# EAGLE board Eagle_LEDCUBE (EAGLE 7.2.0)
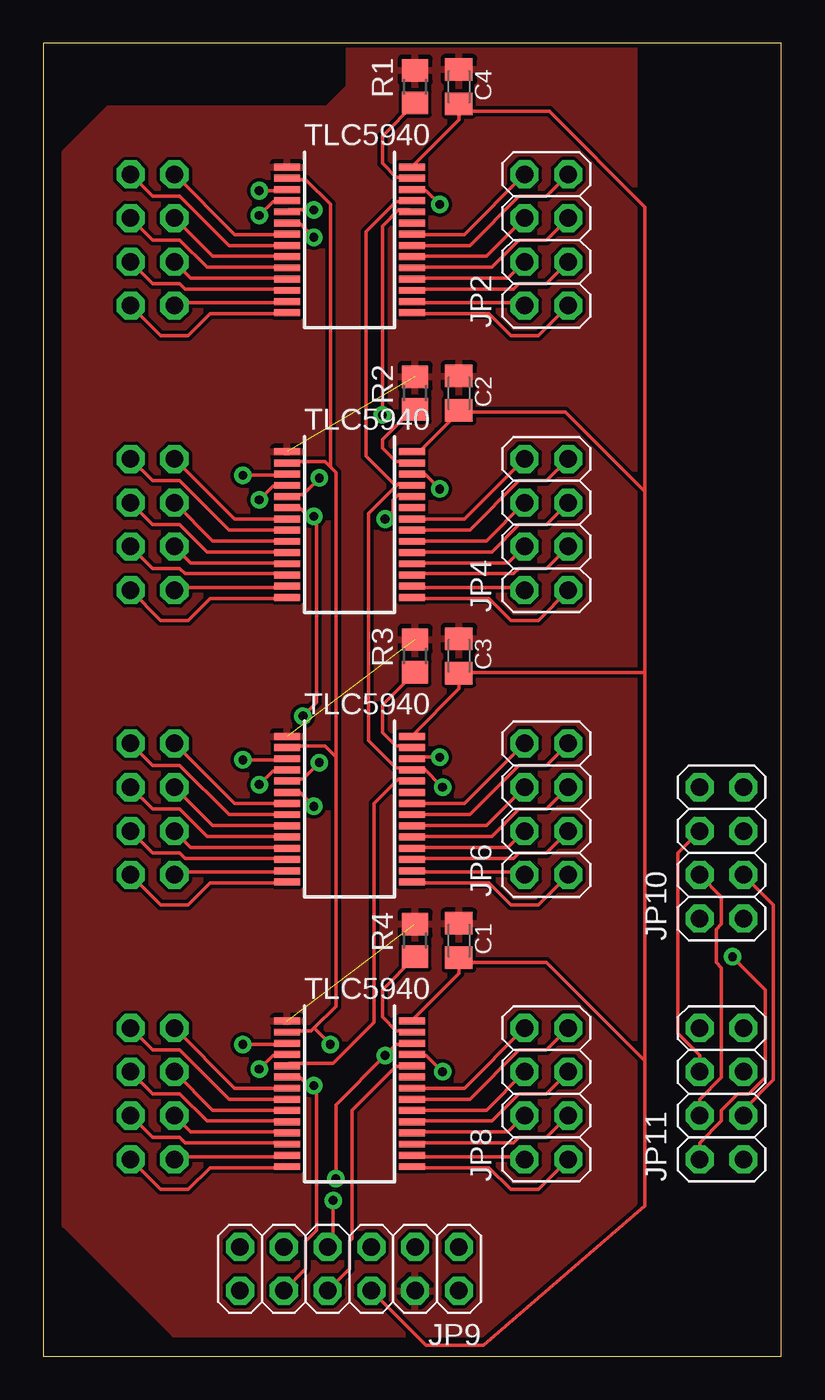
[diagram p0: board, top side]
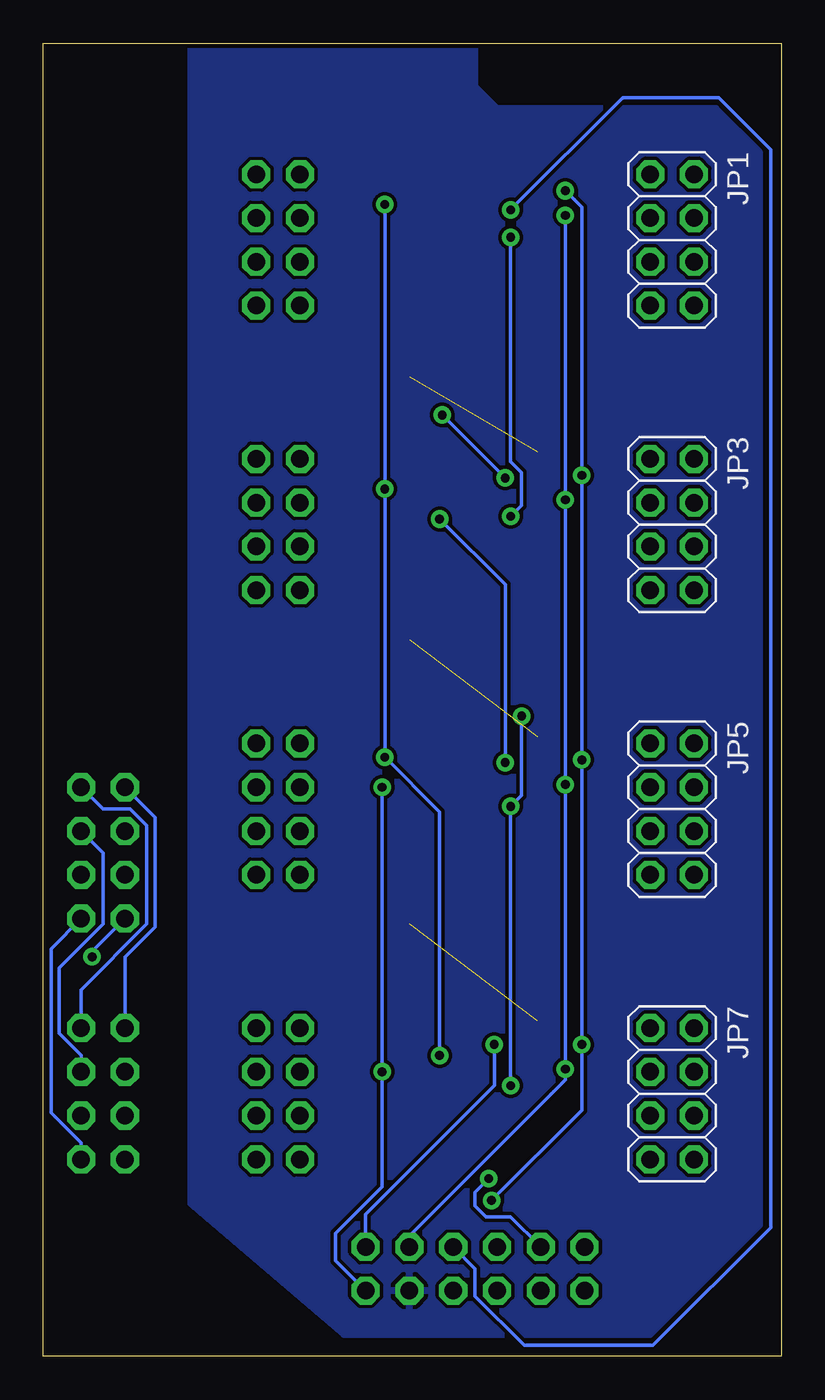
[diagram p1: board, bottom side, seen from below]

Size 42.85 x 76.19 mm. Coordinates in mm from the lower left corner, seen from the top.
Outline: 0,0 42.85,0 42.85,76.19 0,76.19 0,0
Copper layers (1*16): Top 0.035mm / dielectric 1.5mm / Bottom 0.035mm
Design rules "8mils": minimum track width 8mil, minimum drill 20mil, track to track 8mil, track to pad 8mil, pad to pad 8mil, via to via 8mil, smd to smd 8mil, copper to edge 10mil, drill to drill 8mil, minimum pad ring 12mil, minimum via ring 10mil, stop-mask expansion 4mil, vias tented up to drill 25mil, thermal gap 10mil

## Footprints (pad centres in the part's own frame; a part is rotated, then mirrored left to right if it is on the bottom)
C0805K = smd 1.3 x 1.6: 1 -1,0; 2 1,0
IC-SSOP28 = smd 0.4 x 1.5: 1 -4.225,-3.625; 2 -3.575,-3.625; 3 -2.925,-3.625; 4 -2.275,-3.625; 5 -1.625,-3.625; 6 -0.975,-3.625; 7 -0.325,-3.625; 8 0.325,-3.625; 9 0.975,-3.625; 10 1.625,-3.625; 11 2.275,-3.625; 12 2.925,-3.625; 13 3.575,-3.625; 14 4.225,-3.625; 15 4.225,3.625; 16 3.575,3.625; 17 2.925,3.625; 18 2.275,3.625; 19 1.625,3.625; 20 0.975,3.625; 21 0.325,3.625; 22 -0.325,3.625; 23 -0.975,3.625; 24 -1.625,3.625; 25 -2.275,3.625; 26 -2.925,3.625; 27 -3.575,3.625; 28 -4.225,3.625
2X04 = drill 1.016 octagon: 1 -3.81,-1.27; 2 -3.81,1.27; 3 -1.27,-1.27; 4 -1.27,1.27; 5 1.27,-1.27; 6 1.27,1.27; 7 3.81,-1.27; 8 3.81,1.27
2X06 = drill 1.016 octagon: 1 -6.35,-1.27; 2 -6.35,1.27; 3 -3.81,-1.27; 4 -3.81,1.27; 5 -1.27,-1.27; 6 -1.27,1.27; 7 1.27,-1.27; 8 1.27,1.27; 9 3.81,-1.27; 10 3.81,1.27; 11 6.35,-1.27; 12 6.35,1.27
R0805 = smd 1.3 x 1.5: 1 -0.95,0; 2 0.95,0

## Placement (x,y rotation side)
C1  [C0805K]  24.13,24.13 270 top
C2  [C0805K]  24.13,55.88 270 top
C3  [C0805K]  24.13,40.64 270 top
C4  [C0805K]  24.13,73.66 270 top
IC1  [IC-SSOP28]  17.78,64.77 270 top
IC2  [IC-SSOP28]  17.78,48.26 270 top
IC3  [IC-SSOP28]  17.78,31.75 270 top
IC4  [IC-SSOP28]  17.78,15.24 270 top
JP1  [2X04]  6.35,64.77 270 bottom
JP2  [2X04]  29.21,64.77 90 top
JP3  [2X04]  6.35,48.26 270 bottom
JP4  [2X04]  29.21,48.26 90 top
JP5  [2X04]  6.35,31.75 270 bottom
JP6  [2X04]  29.21,31.75 90 top
JP7  [2X04]  6.35,15.24 270 bottom
JP8  [2X04]  29.21,15.24 90 top
JP9  [2X06]  17.78,5.08 180 top
JP10  [2X04]  39.37,29.21 90 top
JP11  [2X04]  39.37,15.24 90 top
R1  2.2k  [R0805]  21.59,73.66 90 top
R2  2.2k  [R0805]  21.59,55.88 90 top
R3  2.2k  [R0805]  21.59,40.64 90 top
R4  2.2k  [R0805]  21.59,24.13 90 top

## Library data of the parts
C1-C4 R1-R4 = resistor
IC1-IC4 = TLC5940
JP1-JP11 = pinhead

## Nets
A1: IC1.7 JP1.1
A2: IC1.8 JP1.2
A3: IC1.9 JP1.3
A4: IC1.10 JP1.4
A5: IC1.11 JP1.5
A6: IC1.12 JP1.6
A7: IC1.13 JP1.7
A8: IC1.14 JP1.8
A9: IC1.15 JP2.1
A10: IC1.16 JP2.2
A11: IC1.17 JP2.3
A12: IC1.18 JP2.4
A13: IC1.19 JP2.5
A14: IC1.20 JP2.6
A15: IC1.21 JP2.7
A16: IC1.22 JP2.8
B1: IC2.7 JP3.1
B2: IC2.8 JP3.2
B3: IC2.9 JP3.3
B4: IC2.10 JP3.4
B5: IC2.11 JP3.5
B6: IC2.12 JP3.6
B7: IC2.13 JP3.7
B8: IC2.14 JP3.8
B9: IC2.15 JP4.1
B10: IC2.16 JP4.2
B11: IC2.17 JP4.3
B12: IC2.18 JP4.4
B13: IC2.19 JP4.5
B14: IC2.20 JP4.6
B15: IC2.21 JP4.7
B16: IC2.22 JP4.8
BLANK: IC1.2 IC2.2 IC3.2 IC4.2 JP9.1
C1: IC3.7 JP5.1
C2: IC3.8 JP5.2
C3: IC3.9 JP5.3
C4: IC3.10 JP5.4
C5: IC3.11 JP5.5
C6: IC3.12 JP5.6
C7: IC3.13 JP5.7
C8: IC3.14 JP5.8
C9: IC3.15 JP6.1
C10: IC3.16 JP6.2
C11: IC3.17 JP6.3
C12: IC3.18 JP6.4
C13: IC3.19 JP6.5
C14: IC3.20 JP6.6
C15: IC3.21 JP6.7
C16: IC3.22 JP6.8
D1: IC4.7 JP7.1
D2: IC4.8 JP7.2
D3: IC4.9 JP7.3
D4: IC4.10 JP7.4
D5: IC4.11 JP7.5
D6: IC4.12 JP7.6
D7: IC4.13 JP7.7
D8: IC4.14 JP7.8
D9: IC4.15 JP8.1
D10: IC4.16 JP8.2
D11: IC4.17 JP8.3
D12: IC4.18 JP8.4
D13: IC4.19 JP8.5
D14: IC4.20 JP8.6
D15: IC4.21 JP8.7
D16: IC4.22 JP8.8
DCPRG: IC1.26 IC2.26 IC3.26 IC4.26 JP9.9
GND: C1.1 C2.1 C3.1 C4.1 IC1.1 IC2.1 IC3.1 IC4.1 JP9.4 R1.2 R2.2 R3.2 R4.2
GSCLK: IC1.25 IC2.25 IC3.25 IC4.25 JP9.2
L1: JP10.1 JP11.1
L2: JP10.2 JP11.2
L3: JP10.3 JP11.3
L4: JP10.4 JP11.4
L5: JP10.5 JP11.5
L6: JP10.6 JP11.6
L7: JP10.7 JP11.7
L8: JP10.8 JP11.8
N$5: IC1.27 R1.1
N$16: IC2.27 R2.1
N$26: IC3.27 R3.1
N$35: IC4.27 R4.1
SCLK: IC1.4 IC2.4 IC3.4 IC4.4 JP9.3
SIN: IC1.5 JP9.5
SIN_B: IC1.24 IC2.5
SIN_C: IC2.24 IC3.5
SIN_D: IC3.24 IC4.5
SIN_E: IC4.24 JP9.8
VCC: C1.2 C2.2 C3.2 C4.2 IC1.28 IC2.28 IC3.28 IC4.28 JP9.6
VPRG: IC1.6 IC2.6 IC3.6 IC4.6 JP9.10
XLAT: IC1.3 IC2.3 IC3.3 IC4.3 JP9.7

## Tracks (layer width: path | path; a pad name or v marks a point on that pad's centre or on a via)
A1
  Top 0.203: JP1.1 11.11,65.09 14.13,65.09 IC1.7
A2
  Top 0.203: JP1.2 6.35,67.31 7.94,67.31 10.79,64.45 14.13,64.45 IC1.8
A3
  Top 0.203: JP1.3 9.84,63.82 14.13,63.82 IC1.9
A4
  Top 0.203: JP1.4 6.35,64.77 7.94,64.77 9.52,63.18 14.13,63.18 IC1.10
A5
  Top 0.203: JP1.5 8.57,62.55 14.13,62.55 IC1.11
A6
  Top 0.203: JP1.6 6.35,62.23 7.94,62.23 8.25,61.91 14.13,61.91 IC1.12
A7
  Top 0.203: JP1.7 7.78,61.12 14.13,61.12 IC1.13
A8
  Top 0.203: JP1.8 6.83,59.21 8.41,59.21 9.68,60.48 14.13,60.48 IC1.14
A9
  Top 0.203: JP2.1 28.73,59.21 27.15,59.21 25.88,60.48 21.43,60.48 IC1.15
A10
  Top 0.203: JP2.2 27.78,61.12 21.43,61.12 IC1.16
A11
  Top 0.203: JP2.3 29.21,62.23 27.62,62.23 27.31,61.91 21.43,61.91 IC1.17
A12
  Top 0.203: JP2.4 26.99,62.55 21.43,62.55 IC1.18
A13
  Top 0.203: JP2.5 29.21,64.77 27.62,64.77 26.04,63.18 21.43,63.18 IC1.19
A14
  Top 0.203: JP2.6 25.72,63.82 21.43,63.82 IC1.20
A15
  Top 0.203: JP2.7 29.21,67.31 27.62,67.31 24.76,64.45 21.43,64.45 IC1.21
A16
  Top 0.203: JP2.8 24.45,65.09 21.43,65.09 IC1.22
B1
  Top 0.203: JP3.1 11.11,48.58 14.13,48.58 IC2.7
B2
  Top 0.203: JP3.2 6.35,50.8 7.94,50.8 10.79,47.94 14.13,47.94 IC2.8
B3
  Top 0.203: JP3.3 9.84,47.31 14.13,47.31 IC2.9
B4
  Top 0.203: JP3.4 6.35,48.26 7.94,48.26 9.52,46.67 14.13,46.67 IC2.10
B5
  Top 0.203: JP3.5 8.57,46.04 14.13,46.04 IC2.11
B6
  Top 0.203: JP3.6 6.35,45.72 7.94,45.72 8.25,45.4 14.13,45.4 IC2.12
B7
  Top 0.203: JP3.7 7.78,44.61 14.13,44.61 IC2.13
B8
  Top 0.203: JP3.8 6.83,42.7 8.41,42.7 9.68,43.97 14.13,43.97 IC2.14
B9
  Top 0.203: JP4.1 28.73,42.7 27.15,42.7 25.88,43.97 21.43,43.97 IC2.15
B10
  Top 0.203: JP4.2 27.78,44.61 21.43,44.61 IC2.16
B11
  Top 0.203: JP4.3 29.21,45.72 27.62,45.72 27.31,45.4 21.43,45.4 IC2.17
B12
  Top 0.203: JP4.4 26.99,46.04 21.43,46.04 IC2.18
B13
  Top 0.203: JP4.5 29.21,48.26 27.62,48.26 26.04,46.67 21.43,46.67 IC2.19
B14
  Top 0.203: JP4.6 25.72,47.31 21.43,47.31 IC2.20
B15
  Top 0.203: JP4.7 29.21,50.8 27.62,50.8 24.76,47.94 21.43,47.94 IC2.21
B16
  Top 0.203: JP4.8 24.45,48.58 21.43,48.58 IC2.22
BLANK  (via drill 0.51)
  Top 0.203: 15.72,19.05 16.99,20.32 16.99,34.77 | 15.72,19.05 15.56,18.89 14.29,18.89 IC4.2 | 16.99,34.77 16.35,35.4 14.29,35.4 IC3.2 | 16.67,51.59 16.99,51.28 16.99,34.77 | 16.67,51.59 16.35,51.91 14.29,51.91 IC2.2 | 16.67,51.59 16.67,66.83 15.24,68.26 14.29,68.26 IC1.2 | 15.72,19.05 v16.67,18.1
  Bottom 0.203: JP9.1 24.13,8.26 16.67,15.72 v16.67,18.1
C1
  Top 0.203: JP5.1 11.11,32.07 14.13,32.07 IC3.7
C2
  Top 0.203: JP5.2 6.35,34.29 7.94,34.29 10.79,31.43 14.13,31.43 IC3.8
C3
  Top 0.203: JP5.3 9.84,30.8 14.13,30.8 IC3.9
C4
  Top 0.203: JP5.4 6.35,31.75 7.94,31.75 9.52,30.16 14.13,30.16 IC3.10
C5
  Top 0.203: JP5.5 8.57,29.53 14.13,29.53 IC3.11
C6
  Top 0.203: JP5.6 6.35,29.21 7.94,29.21 8.25,28.89 14.13,28.89 IC3.12
C7
  Top 0.203: JP5.7 7.78,28.1 14.13,28.1 IC3.13
C8
  Top 0.203: JP5.8 6.83,26.19 8.41,26.19 9.68,27.46 14.13,27.46 IC3.14
C9
  Top 0.203: JP6.1 28.73,26.19 27.15,26.19 25.88,27.46 21.43,27.46 IC3.15
C10
  Top 0.203: JP6.2 27.78,28.1 21.43,28.1 IC3.16
C11
  Top 0.203: JP6.3 29.21,29.21 27.62,29.21 27.31,28.89 21.43,28.89 IC3.17
C12
  Top 0.203: JP6.4 26.99,29.53 21.43,29.53 IC3.18
C13
  Top 0.203: JP6.5 29.21,31.75 27.62,31.75 26.04,30.16 21.43,30.16 IC3.19
C14
  Top 0.203: JP6.6 25.72,30.8 21.43,30.8 IC3.20
C15
  Top 0.203: JP6.7 29.21,34.29 27.62,34.29 24.76,31.43 21.43,31.43 IC3.21
C16
  Top 0.203: JP6.8 24.45,32.07 21.43,32.07 IC3.22
D1
  Top 0.203: JP7.1 11.11,15.56 14.13,15.56 IC4.7
D2
  Top 0.203: JP7.2 6.35,17.78 7.94,17.78 10.79,14.92 14.13,14.92 IC4.8
D3
  Top 0.203: JP7.3 9.84,14.29 14.13,14.29 IC4.9
D4
  Top 0.203: JP7.4 6.35,15.24 7.94,15.24 9.52,13.65 14.13,13.65 IC4.10
D5
  Top 0.203: JP7.5 8.57,13.02 14.13,13.02 IC4.11
D6
  Top 0.203: JP7.6 6.35,12.7 7.94,12.7 8.25,12.38 14.13,12.38 IC4.12
D7
  Top 0.203: JP7.7 7.78,11.59 14.13,11.59 IC4.13
D8
  Top 0.203: JP7.8 6.83,9.68 8.41,9.68 9.68,10.95 14.13,10.95 IC4.14
D9
  Top 0.203: JP8.1 28.73,9.68 27.15,9.68 25.88,10.95 21.43,10.95 IC4.15
D10
  Top 0.203: JP8.2 27.78,11.59 21.43,11.59 IC4.16
D11
  Top 0.203: JP8.3 29.21,12.7 27.62,12.7 27.31,12.38 21.43,12.38 IC4.17
D12
  Top 0.203: JP8.4 26.99,13.02 21.43,13.02 IC4.18
D13
  Top 0.203: JP8.5 29.21,15.24 27.62,15.24 26.04,13.65 21.43,13.65 IC4.19
D14
  Top 0.203: JP8.6 25.72,14.29 21.43,14.29 IC4.20
D15
  Top 0.203: JP8.7 29.21,17.78 27.62,17.78 24.76,14.92 21.43,14.92 IC4.21
D16
  Top 0.203: JP8.8 24.45,15.56 21.43,15.56 IC4.22
DCPRG  (via drill 0.51)
  Top 0.203: v16.99,10.32 16.99,14.61 v19.84,17.46 20.48,18.1 21.27,18.1 IC4.26 | v23.02,34.77 21.43,34.77 IC3.26 | v23.02,50.32 22.07,51.28 21.43,51.28 IC2.26 | v23.02,66.83 22.22,67.63 21.43,67.63 IC1.26
  Bottom 0.203: v16.99,10.32 17.78,9.53 17.78,8.73 17.14,8.1 15.72,8.1 JP9.9 | v23.02,66.83 v23.02,50.32 v23.02,34.77 19.84,31.59 v19.84,17.46
GND  (3 unrouted)
  pour Bottom: 1.27,7.62 1.27,69.85 3.81,72.39 16.51,72.39 17.78,73.66 17.78,76.2 34.29,76.2 34.29,8.89 25.4,1.27 7.62,1.27
  pour Top: 1.27,7.62 1.27,69.85 3.81,72.39 16.51,72.39 17.78,73.66 17.78,76.2 34.29,76.2 34.29,8.89 25.4,1.27 7.62,1.27
GSCLK  (via drill 0.51)
  Top 0.203: v23.18,16.51 22.22,17.46 21.43,17.46 IC4.25 | 20.48,50.48 20.64,50.64 21.27,50.64 IC2.25 | 20.48,50.48 18.89,48.9 18.89,35.72 20.48,34.13 21.27,34.13 IC3.25 21.43,34.13 22.07,34.13 v23.18,33.02 | 20.48,50.48 18.73,52.23 18.73,65.25 20.48,66.99 21.27,66.99 IC1.25
  Bottom 0.203: JP9.2 25.88,5.56 25.88,7.14 23.18,9.84 v23.18,16.51 v23.18,33.02
L1
  Bottom 0.203: JP11.1 40.64,12.38 42.39,14.13 42.39,23.65 JP10.1
L2  (via drill 0.51)
  Top 0.203: JP11.2 38.1,12.38 39.37,13.65 39.37,14.29 40.32,15.24 40.96,15.24 41.91,16.19 41.91,21.27 v40,23.18
  Bottom 0.203: v40,23.18 40,23.5 JP10.2
L3
  Top 0.203: JP11.3 40.64,14.29 42.39,16.03 42.39,26.19 JP10.3
L4
  Top 0.203: JP11.4 38.1,14.92 39.37,16.19 39.37,22.54 39.05,22.86 39.05,24.77 39.37,25.08 39.37,26.67 JP10.4
L5
  Bottom 0.203: JP11.5 40.64,17.46 41.91,18.73 41.91,22.54 39.37,25.08 39.37,29.21 JP10.5
L6
  Top 0.203: JP11.6 38.1,17.46 36.83,18.73 36.83,29.21 JP10.6
L7
  Bottom 0.203: JP11.7 40.64,21.27 36.83,25.08 36.83,30.8 37.78,31.75 39.37,31.75 JP10.7
L8
  Bottom 0.203: JP11.8 38.1,23.18 36.35,24.92 36.35,31.27 JP10.8
N$5
  Top 0.203: IC1.27 21.27,68.42 20.48,68.42 19.68,69.22 19.68,70.8 R1.1
N$16
  Top 0.203: IC2.27 21.27,51.91 20.48,51.91 19.68,52.7 19.68,53.18 21.59,55.09 R2.1
N$26
  Top 0.203: IC3.27 21.27,35.4 20.48,35.4 19.68,36.2 19.68,37.78 R3.1
N$35
  Top 0.203: IC4.27 21.27,18.89 20.48,18.89 19.68,19.68 19.68,21.27 R4.1
SCLK  (via drill 0.51)
  Top 0.203: v12.54,16.67 13.34,17.46 14.13,17.46 IC4.4 | v12.54,33.18 13.34,33.97 14.13,33.97 IC3.4 | v12.54,49.69 13.34,50.48 14.13,50.48 IC2.4 | v12.54,66.2 13.34,66.99 14.13,66.99 IC1.4
  Bottom 0.203: JP9.3 21.59,6.99 12.54,16.03 v12.54,16.67 v12.54,33.18 v12.54,49.69 v12.54,66.2
SIN  (via drill 0.51)
  Top 0.203: v15.72,66.52 14.29,66.52 IC1.5
  Bottom 0.203: v15.72,66.52 9.21,73.03 3.65,73.03 0.63,70.01 0.63,7.46 7.46,0.64 14.92,0.64 17.78,3.49 17.78,5.08 JP9.5
SIN_B  (via drill 0.51)
  Top 0.203: v16.03,50.96 15.08,50.01 14.29,50.01 IC2.5 | v19.68,54.61 19.68,65.56 20.64,66.52 21.27,66.52 IC1.24
  Bottom 0.203: v19.68,54.61 v16.03,50.96
SIN_C  (via drill 0.51)
  Top 0.203: v16.03,34.45 15.08,33.5 14.29,33.5 IC3.5 | v19.84,48.58 20.32,49.05 20.32,49.69 20.64,50.01 21.27,50.01 IC2.24
  Bottom 0.203: v16.03,34.45 16.03,44.77 v19.84,48.58
SIN_D
  Top 0.203: IC4.5 14.29,16.99 16.83,16.99 19.21,19.37 19.21,32.07 20.64,33.5 21.27,33.5 IC3.24
SIN_E
  Top 0.203: JP9.8 17.78,5.08 17.78,6.67 17.94,6.83 17.94,14.29 20.48,16.83 21.27,16.83 IC4.24
VCC
  Top 0.203: 24.13,72.23 C4.2 24.13,72.55 | 24.13,72.23 24.13,71.75 21.43,69.06 IC1.28 | IC3.28 21.43,36.04 24.13,38.73 C3.2 24.13,39.69 34.92,39.69 | 24.13,54.77 21.91,52.55 21.43,52.55 IC2.28 | 24.13,22.86 C1.2 24.13,23.02 | 24.13,22.86 24.13,22.23 21.43,19.53 IC4.28 | JP9.6 22.22,0.64 25.56,0.64 34.92,8.73 34.92,17.14 | 34.92,17.14 29.21,22.86 24.13,22.86 | 24.13,54.77 30.32,54.77 34.92,50.16 | 34.92,17.14 34.92,39.69 | 34.92,39.69 34.92,50.16 | 24.13,54.77 C2.2 | 24.13,72.23 29.37,72.23 34.92,66.67 34.92,50.16
VPRG  (via drill 0.51)
  Top 0.203: 15.56,15.56 15.88,15.24 15.88,7.3 15.24,6.67 15.24,5.08 JP9.10 | 15.56,15.56 14.92,16.19 14.29,16.19 IC4.6 | v15.72,31.91 14.92,32.7 14.29,32.7 IC3.6 | 15.56,15.56 v15.72,15.72 | 15.56,48.58 15.88,48.26 15.88,37.94 v15.08,37.15 | 15.56,48.58 14.92,49.21 14.29,49.21 IC2.6 | v15.72,64.93 14.92,65.72 14.29,65.72 IC1.6 | 15.56,48.58 v15.72,48.74
  Bottom 0.203: v15.72,15.72 v15.72,31.91 15.08,32.54 v15.08,37.15 | v15.72,64.93 15.72,51.91 15.08,51.28 15.08,49.37 v15.72,48.74
XLAT  (via drill 0.51)
  Top 0.203: v11.59,18.1 14.13,18.1 IC4.3 | v16.83,9.05 16.83,6.67 JP9.7 | v11.59,34.61 14.13,34.61 IC3.3 | v11.59,51.12 14.13,51.12 IC2.3 | v12.54,67.63 14.13,67.63 IC1.3
  Bottom 0.203: v16.83,9.05 11.59,14.29 v11.59,18.1 v11.59,34.61 v11.59,51.12 11.59,66.67 v12.54,67.63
